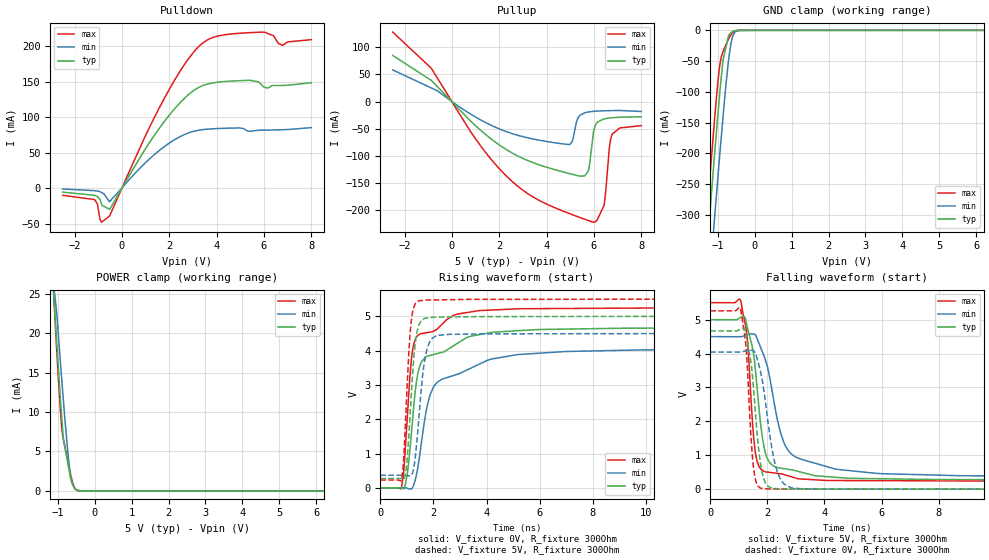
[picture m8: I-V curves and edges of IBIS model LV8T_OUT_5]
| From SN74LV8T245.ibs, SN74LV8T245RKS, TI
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[Model]   LV8T_OUT_5
Model_type   I/O
Polarity   Non-Inverting
Enable   Active-Low
Vinl = 0.8
Vinh = 2
Vmeas = 2.5
Vref = 0
Cref = 2pF
Rref = 100000
|   typ   min   max
C_comp   6.7pF   6.5pF   7pF
[Voltage Range]   5   4.5   5.5
[Temperature Range]   25   125   -40
[Pullup Reference]   5   4.5   5.5
[Pulldown Reference]   0   0   0
[Power Clamp Reference]   5   4.5   5.5
[GND Clamp Reference]   0   0   0
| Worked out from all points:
|   slope of the pulldown table from 0 to 0.75 V, typ, clamps not added: 17.8 ohm
|   slope of the pullup table from 0 to 0.75 V, typ, clamps not added: 22 ohm
|   GND clamp passes 1 mA (typ) near -0.55 V on its own axis
|   POWER clamp passes 1 mA (typ) near -0.61 V on its own axis
|   falling waveform, V_fixture 5V, R_fixture 300Ohm: 20-80 % time 387ps typ, 706ps min, 255ps max; typ from 5 V to 0.271 V
|   rising waveform, V_fixture 0V, R_fixture 300Ohm: 20-80 % time 525ps typ, 1.14ns min, 332ps max; typ from 0 V to 4.67 V
|   rising waveform, V_fixture 5V, R_fixture 300Ohm: 20-80 % time 248ps typ, 306ps min, 208ps max; typ from 0.271 V to 5 V
|   falling waveform, V_fixture 0V, R_fixture 300Ohm: 20-80 % time 305ps typ, 437ps min, 216ps max; typ from 4.67 V to 0 V
[Pulldown]
|   Voltage   I(typ)   I(min)   I(max)
-2.5V     -5.66mA    -1.23mA    -10.11mA
-1.156V   -10.12mA   -3.592mA   -16.15mA
-1.04V    -11.78mA   -4.168mA   -22.05mA
-862mV    -22.47mA   -6.167mA   -48.08mA
-515.5mV  -30.04mA   -18.87mA   -39.04mA
1.942V    100.4mA    62.15mA    135.9mA
2.876V    133.8mA    78.69mA    185.5mA
3.622V    147mA      83.26mA    209.4mA
5.407V    152.2mA    80.2mA     219.4mA
5.963V    143.4mA    81.82mA    220.2mA
6.782V    145mA      82.43mA    201.6mA
8V        148.7mA    85.37mA    209.6mA
[GND Clamp]
|   Voltage   I(typ)   I(min)   I(max)
-2.5V     -1.32A     -1.415A    -1.27A
-1.335V   -392.6mA   -495.4mA   -334.5mA
-1.23V    -311.6mA   -414.9mA   -253.3mA
-1.093V   -208.7mA   -311.7mA   -151.2mA
-956.5mV  -111.2mA   -211.8mA   -63.42mA
-904mV    -76.9mA    -174.2mA   -43.79mA
-851.5mV  -47.24mA   -138.5mA   -33.82mA
-704.5mV  -8.389mA   -48.27mA   -13.86mA
-631mV    -3.534mA   -18.64mA   -6.616mA
-589mV    -1.77mA    -9.001mA   -3.449mA
-421mV    -89.14uA   -161.4uA   -117.3uA
8V        0A         0A         0A
[Pullup]
|   Voltage   I(typ)   I(min)   I(max)
-2.5V     84.58mA    58.02mA    127.5mA
-872.5mV  38.8mA     24.88mA    61.23mA
2.277V    -87.61mA   -54.95mA   -135.8mA
5.133V    -134.2mA   -64.93mA   -208.6mA
5.312V    -136mA     -31.31mA   -211.4mA
5.753V    -128.4mA   -19.31mA   -218.3mA
5.984V    -54.52mA   -18.1mA    -221.6mA
6.11V     -39.86mA   -17.7mA    -218.8mA
6.425V    -31.9mA    -17.07mA   -190.8mA
6.656V    -30.19mA   -16.79mA   -83.32mA
6.761V    -29.73mA   -16.69mA   -60.74mA
8V        -27.99mA   -18.28mA   -44.35mA
[POWER Clamp]
|   Voltage   I(typ)   I(min)   I(max)
-2.5V     108.8mA    88.15mA    134mA
-1.135V   27.14mA    27.18mA    27.27mA
-1.051V   20.74mA    23.66mA    19.89mA
-1.02V    18.39mA    22.17mA    17.29mA
-925mV    11.6mA     16.24mA    10.18mA
-883mV    8.872mA    13.69mA    7.695mA
-841mV    6.433mA    11.23mA    6.472mA
-725.5mV  3.503mA    4.969mA    3.854mA
-652mV    1.638mA    1.908mA    2.187mA
-536.5mV  280.5uA    367.5uA    311.9uA
-442mV    20.33uA    85.92uA    9.604uA
8V        0A         0A         0A
[Ramp]
R_load = 300
|   typ   min   max
dV/dt_r   2.80005/5.07819e-10   2.42656/1.15288e-09   3.15563/3.31337e-10
dV/dt_f   2.8373/3.84473e-10   2.47987/7.04948e-10   3.16307/2.52606e-10
[Falling Waveform]
V_fixture = 5V
V_fixture_min = 4.5V
V_fixture_max = 5.5V
R_fixture = 300Ohm
C_fixture = 0F
|   Time   V(typ)   V(min)   V(max)
0s        5V         4.499V     5.5V
1.059ns   5.062V     4.495V     5.58V
1.297ns   4.777V     4.554V     4.45V
1.478ns   4.168V     4.575V     1.975V
1.575ns   3.586V     4.561V     1.115V
1.875ns   1.285V     3.944V     528.8mV
2.56ns    607.6mV    1.414V     436.4mV
3.16ns    506.4mV    889.3mV    301.4mV
5.832ns   308.5mV    464.8mV    250.8mV
15ns      270.7mV    366.1mV    228mV
[Rising Waveform]
V_fixture = 0V
V_fixture_min = 0V
V_fixture_max = 0V
R_fixture = 300Ohm
C_fixture = 0F
|   Time   V(typ)   V(min)   V(max)
0s        78.51uV    150uV      47.34uV
800.9ps   -5.72mV    4.104mV    11.81mV
1.005ns   341.9mV    -8.216mV   1.902V
1.159ns   1.476V     -31.22mV   3.648V
1.315ns   2.805V     227.9mV    4.325V
1.498ns   3.575V     1.028V     4.483V
1.877ns   3.858V     2.714V     4.537V
2.74ns    4.13V      3.27V      5.017V
5.146ns   4.577V     3.881V     5.214V
15ns      4.667V     4.044V     5.259V
[Rising Waveform]
V_fixture = 5V
V_fixture_min = 4.5V
V_fixture_max = 5.5V
R_fixture = 300Ohm
C_fixture = 0F
|   Time   V(typ)   V(min)   V(max)
0s        270.7mV    366.1mV    228mV
803.4ps   264.6mV    368.3mV    253.6mV
879.7ps   245.1mV    368.5mV    818.8mV
985.4ps   617.6mV    363.5mV    2.541V
1.144ns   2.412V     347.9mV    4.686V
1.275ns   3.905V     643.2mV    5.287V
1.426ns   4.673V     1.782V     5.44V
1.7ns     4.942V     3.847V     5.47V
2.148ns   4.972V     4.439V     5.476V
15ns      5V         4.499V     5.5V
[Falling Waveform]
|Gnd
V_fixture = 0V
V_fixture_min = 0V
V_fixture_max = 0V
R_fixture = 300Ohm
C_fixture = 0F
|   Time   V(typ)   V(min)   V(max)
0s        4.667V     4.045V     5.259V
1.059ns   4.72V      4.043V     5.32V
1.257ns   4.535V     4.082V     4.146V
1.418ns   3.777V     4.1V       1.649V
1.504ns   3.085V     4.081V     715.7mV
1.747ns   828.9mV    3.506V     35.8mV
1.947ns   162.1mV    2.475V     12.79mV
2.264ns   20.22mV    765mV      5.857mV
2.799ns   6.522mV    54.25mV    2.768mV
15ns      78.79uV    150.8uV    47.49uV
